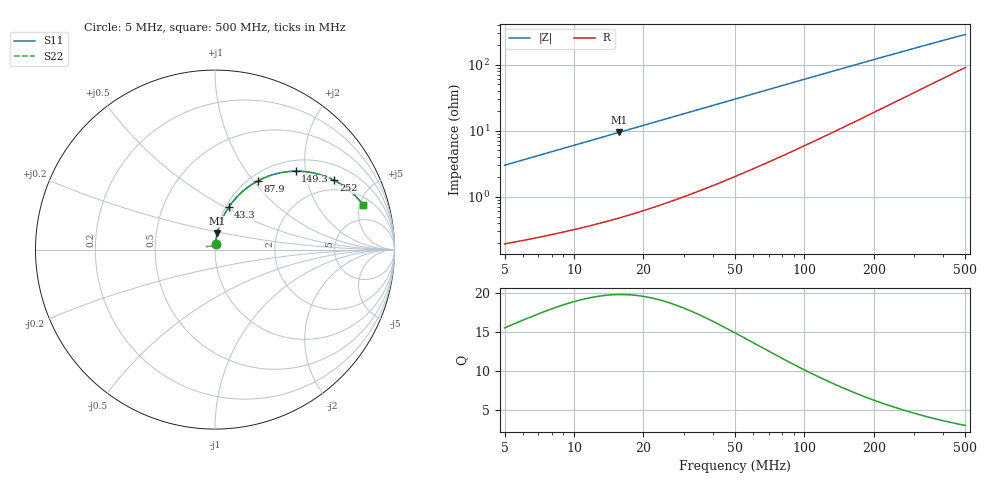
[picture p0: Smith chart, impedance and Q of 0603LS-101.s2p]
# MHz S MA R 50
!Freq  MagS11  AngS11  MagS21  AngS21  MagS12  AngS12  MagS22  AngS22
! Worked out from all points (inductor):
!   801 points, 5 MHz to 500 MHz, reference 50 ohm
!   read as one part in series: L = 95 nH near 5.116 MHz
!   highest Q = 19.8 at 15.63 MHz (marker M1), where L = 95.2 nH
!   S11 on the Smith chart (normalised r, x): 5 MHz: 1.00, +0.06; 43.3 MHz: 1.03, +0.52; 87.9 MHz: 1.10, +1.05; 149.3 MHz: 1.23, +1.77; 252 MHz: 1.56, +2.93; 500 MHz: 2.80, +5.42
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5  0.02982 84.6  0.9976 -1.7  0.9976 -1.7  0.02982 84.6
7.022148  0.04185 84.3  0.9967 -2.4  0.9967 -2.4  0.04185 84.3
9.364185  0.05576 83.7  0.9955 -3.2  0.9955 -3.2  0.05576 83.7
12.2031  0.07257 82.9  0.9936 -4.2  0.9936 -4.2  0.07257 82.9
15.6304  0.09277 81.8  0.991 -5.3  0.991 -5.3  0.09277 81.8
20.84347  0.1232 80.0  0.9861 -7.1  0.9861 -7.1  0.1232 80.0
27.16252  0.1594 77.7  0.9786 -9.2  0.9786 -9.2  0.1594 77.7
34.59155  0.2009 75.1  0.9681 -11.6  0.9681 -11.6  0.2009 75.1
43.29822  0.2477 72.1  0.9534 -14.3  0.9534 -14.3  0.2477 72.1
52.65868  0.2955 68.9  0.9352 -17.1  0.9352 -17.1  0.2955 68.9
62.94627  0.3447 65.6  0.9131 -20.1  0.9131 -20.1  0.3447 65.6
74.81178  0.3971 61.9  0.8855 -23.3  0.8855 -23.3  0.3971 61.9
87.89618  0.4494 58.2  0.8534 -26.6  0.8534 -26.6  0.4494 58.2
115.8697  0.5428 51.1  0.7832 -32.7  0.7832 -32.7  0.5428 51.1
149.2691  0.6264 44.2  0.7033 -38.4  0.7033 -38.4  0.6264 44.2
170.4002  0.667 40.6  0.6571 -41.3  0.6571 -41.3  0.667 40.6
209.638  0.7238 35.0  0.5817 -45.6  0.5817 -45.6  0.7238 35.0
252.0403  0.7664 30.4  0.5145 -48.8  0.5145 -48.8  0.7664 30.4
253.4954  0.7676 30.2  0.5125 -48.9  0.5125 -48.9  0.7676 30.2
336.1012  0.8176 23.8  0.4158 -52.7  0.4158 -52.7  0.8176 23.8
418.2828  0.8455 19.6  0.3495 -54.4  0.3495 -54.4  0.8455 19.6
500  0.8625 16.7  0.3022 -54.9  0.3022 -54.9  0.8625 16.7
